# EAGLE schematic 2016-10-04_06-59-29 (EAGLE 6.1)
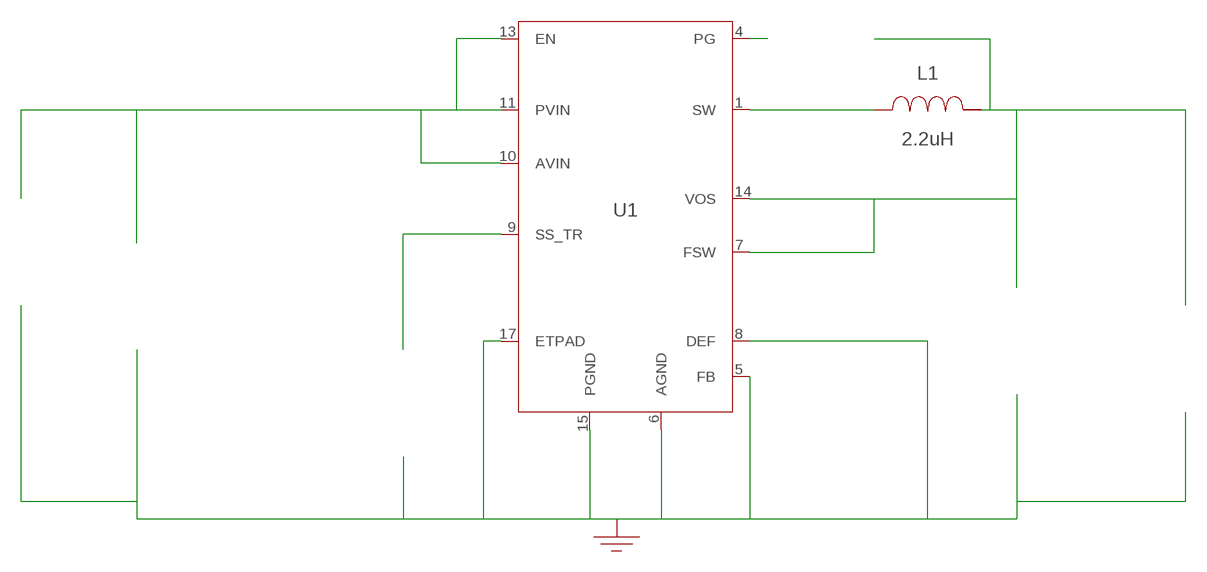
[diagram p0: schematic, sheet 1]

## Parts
CIN  10uF  TMK316BJ106KL-TTMK316BJ106KL-T  [1206]  (not placed on a sheet)
COUT  22uF  GRM21BR60J226ME39LGRM21BR60J226ME39L  [0805]  (not placed on a sheet)
CSS  390pF  CC0805KRX7R9BB391CC0805KRX7R9BB391  [0805]  (not placed on a sheet)
GND  WB_GND  WB_GNDWB_GND  [WB_GND]
IOUT  WB_CURRENT_LOAD  WB_CURRENT_LOADWB_CURRENT_LOAD  [WB_CURRENT_LOAD]  (not placed on a sheet)
L1  2.2uH  IHLP1212BZER2R2M11IHLP1212BZER2R2M11  [IHLP-1212BZ]
RPG  100k  ERJ-6ENF1003VERJ-6ENF1003V  [0805]  (not placed on a sheet)
U1  TPS62152RGTR  TPS62152RGTRTPS62152RGTR  [S-PVQFN-N16]
VIN  WB_BATTERY  WB_BATTERYWB_BATTERY  [WB_BATTERY]  (not placed on a sheet)

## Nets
0: Cin.2@2 Cout.2@2 Css.2@2 GND.1 Iout.-@2 U1.5(FB) U1.6(AGND) U1.8(DEF) U1.15(PGND) U1.16(PGND) U1.17(ETPAD) Vin.-@2
1: Css.1@1 U1.9(SS_TR)
2: Cout.1@1 Iout.+@1 L1.2 Rpg.1@1 U1.7(FSW) U1.14(VOS)
3: Cin.1@1 U1.10(AVIN) U1.11(PVIN) U1.12(PVIN) U1.13(EN) Vin.+@1
4: Rpg.2@2 U1.4(PG)
5: L1.1 U1.1(SW) U1.2(SW) U1.3(SW)
Unconnected: CIN.1 CIN.2 COUT.1 COUT.2 CSS.1 CSS.2 IOUT.1(+) IOUT.2(-) RPG.1 RPG.2 VIN.1(+) VIN.2(-)

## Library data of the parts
CIN = AcceleratedDesigns_Lib:TMK316BJ106KL-T; Cap: 1.0E-5; ESR: 0.0; IRMS: 0.0; Manufacturer_Name: Taiyo Yuden; Manufacturer_Part_Number: TMK316BJ106KL-T; VDC: 25.0; Vendor: Taiyo Yuden
COUT = AcceleratedDesigns_Lib:GRM21BR60J226ME39L; Cap: 2.2E-5; ESR: 0.0; IRMS: 0.0; Manufacturer_Name: MuRata; Manufacturer_Part_Number: GRM21BR60J226ME39L; VDC: 6.3; Vendor: MuRata
CSS = AcceleratedDesigns_Lib:CC0805KRX7R9BB391; Cap: 3.9E-10; ESR: 0.0; IRMS: 0.0; Manufacturer_Name: Yageo America; Manufacturer_Part_Number: CC0805KRX7R9BB391; VDC: 50.0; Vendor: Yageo America
GND = AcceleratedDesigns_Lib:WB_GND; Manufacturer_Name: WB_GND; Manufacturer_Part_Number: WB_GND; PowerPortType: POWER_GROUND; Value: Value
IOUT = AcceleratedDesigns_Lib:WB_CURRENT_LOAD; Manufacturer_Name: WB_CURRENT_LOAD; Manufacturer_Part_Number: WB_CURRENT_LOAD; PowerPortType: POWER_GROUND; Value: Value
L1 = AcceleratedDesigns_Lib:IHLP1212BZER2R2M11; DCR: 46.0; Datasheet_URL: http://www.vishay.com/docs/34289/lp12bz11.pdf; Description: Unknown; IDC: 3.0; L: 2.2E-6; Manufacturer: Vishay; Manufacturer_Name: Vishay-Dale; Manufacturer_Part_Number: IHLP1212BZER2R2M11; PACKAGE_DESIGNATOR: IHLP-1212BZ; Vendor: Vishay-Dale
RPG = AcceleratedDesigns_Lib:ERJ-6ENF1003V; Manufacturer_Name: Panasonic; Manufacturer_Part_Number: ERJ-6ENF1003V; Power: 0.125; Resistance: 100000.0; Tolerance: 1.0; Vendor: Panasonic
U1 = AcceleratedDesigns_Lib:TPS62152RGTR; Datasheet_URL: http://www.ti.com/product/tps62131; Frequency: 2500000.0; Imax: 3.0; Manufacturer_Name: Texas Instruments; Manufacturer_Part_Number: TPS62131RGTR; Mktg_Package: S-PVQFN-N16; NSID: TPS62131RGTR; Package: S-PVQFN-N16; Vendor: Texas Instruments
VIN = AcceleratedDesigns_Lib:WB_BATTERY; Manufacturer_Name: WB_BATTERY; Manufacturer_Part_Number: WB_BATTERY; PowerPortType: POWER_GROUND; Value: Value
